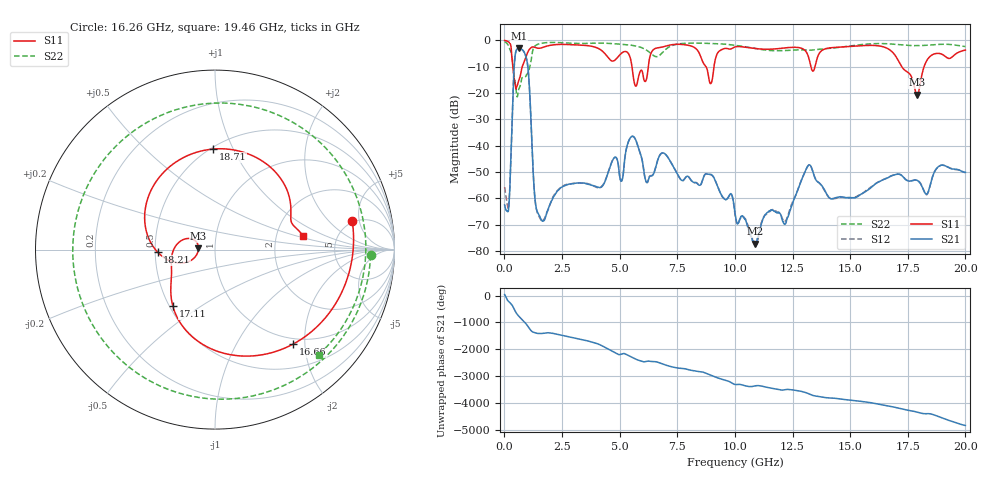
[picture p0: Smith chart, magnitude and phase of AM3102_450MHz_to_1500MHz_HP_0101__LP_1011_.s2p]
!Agilent Technologies,E8364B,MY43040894,A.07.50.67
!Agilent E8364B: A.07.50.67
!Date: Thursday, January 11, 2018 05:42:42
!Correction: S11(Full 2 Port(1,2))
!S21(Full 2 Port(1,2))
!S12(Full 2 Port(1,2))
!S22(Full 2 Port(1,2))
!S2P File: Measurements: S11, S21, S12, S22:
# Hz S  dB  R 50
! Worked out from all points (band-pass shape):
!   1601 points, 10 MHz to 20 GHz, reference 50 ohm
!   highest |S21| = -3.11 dB at 634.7 MHz (marker M1); lowest = -77.3 dB at 10.89 GHz (marker M2)
!   |S21| within 3 dB of the highest: 462.9 MHz to 931.6 MHz (468.7 MHz wide, 67.2 % of centre)
!   lowest |S11| = -20.7 dB at 17.9 GHz (marker M3), VSWR 1.20, Z = 41.6 + j0.597 ohm
!   |S11| at or under -10 dB: 365.5 MHz to 776.5 MHz (411.1 MHz wide, 72 % of centre); 5.536 GHz to 6.242 GHz (706.8 MHz wide, 12 % of centre); 17.24 GHz to 18.21 GHz (971.3 MHz wide, 5.48 % of centre)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
!   |S22| runs from -21.5 to -0.5 dB; largest |S21 - S12| = 0.0019
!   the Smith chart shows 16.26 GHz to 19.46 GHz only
!   S11 on the Smith chart (normalised r, x): 16.26 GHz: 4.77, +3.96; 16.66 GHz: 0.89, -1.76; 17.11 GHz: 0.52, -0.39; 18.21 GHz: 0.51, -0.02; 18.71 GHz: 0.51, +0.84; 19.46 GHz: 2.86, +0.58
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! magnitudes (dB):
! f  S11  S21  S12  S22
! 10 MHz  -0.1  -62.5  -55.8  -0.5
! 184.9 MHz  -0.6  -64.0  -63.0  -2.2
! 447.3 MHz  -15.7  -7.5  -7.5  -14.9
! 634.7 MHz  -15.0  -3.1  -3.1  -18.3
! 997 MHz  -4.9  -8.7  -8.7  -12.8
! 1.309 GHz  -2.6  -58.5  -58.7  -2.3
! 1.522 GHz  -3.0  -66.6  -67.2  -1.3
! 3.346 GHz  -1.9  -54.2  -54.2  -1.2
! 5.707 GHz  -17.4  -38.0  -38.0  -2.2
! 6.682 GHz  -2.8  -44.8  -44.7  -6.0
! 10.01 GHz  -2.5  -65.6  -66.2  -1.9
! 10.89 GHz  -3.1  -77.3  -78.0  -3.1
! 13.34 GHz  -11.3  -48.8  -48.8  -3.7
! 16.26 GHz  -2.1  -53.7  -53.6  -1.2
! 16.66 GHz  -3.3  -52.1  -52.0  -1.3
! 16.68 GHz  -3.4  -52.0  -51.9  -1.3
! 17.11 GHz  -8.1  -50.8  -50.9  -1.6
! 17.9 GHz  -20.7  -53.2  -53.1  -2.0
! 18.21 GHz  -9.9  -57.4  -57.5  -1.9
! 18.71 GHz  -5.0  -49.1  -49.1  -1.6
! 19.46 GHz  -6.0  -48.9  -48.9  -1.7
! 20 GHz  -3.7  -50.2  -50.2  -2.4
